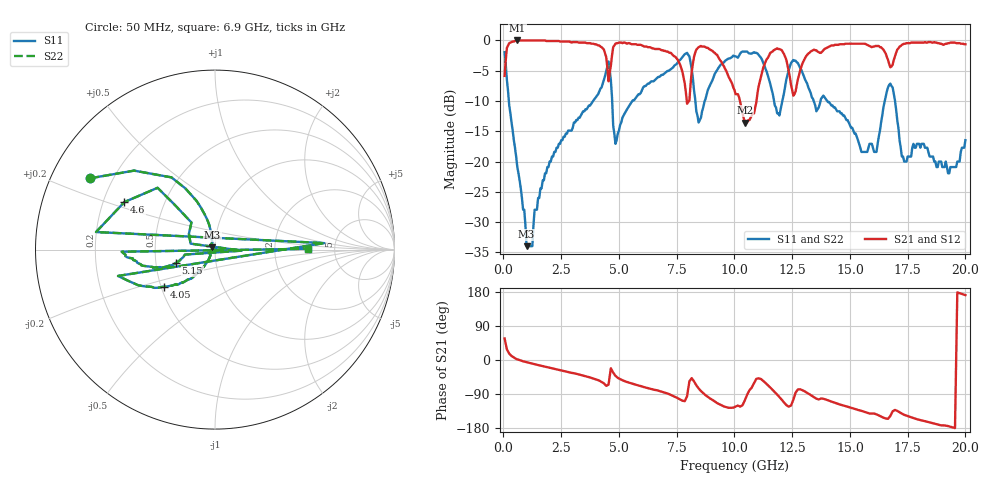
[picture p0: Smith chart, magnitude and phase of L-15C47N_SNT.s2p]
# MHZ S MA R 50
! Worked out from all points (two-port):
!   400 points, 50 MHz to 20 GHz, reference 50 ohm
!   highest |S21| = 0.00 dB at 600 MHz (marker M1); lowest = -13.6 dB at 10.45 GHz (marker M2)
!   |S21| within 3 dB of the highest: 105.5 MHz to 4.457 GHz (4.352 GHz wide, 191 % of centre); 13.05 GHz to 16.63 GHz (3.581 GHz wide, 24.1 % of centre)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
!   lowest |S11| = -34.0 dB at 1 GHz (marker M3), VSWR 1.04, Z = 48.5 + j1.27 ohm
!   |S11| at or under -10 dB: 234 MHz to 3.881 GHz (3.647 GHz wide, 177 % of centre); 14.02 GHz to 16.51 GHz (2.492 GHz wide, 16.3 % of centre); 16.95 GHz to end of sweep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
!   |S22| runs from -34.0 to -1.8 dB; largest |S21 - S12| = 0
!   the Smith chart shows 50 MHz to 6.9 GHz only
!   S11 on the Smith chart (normalised r, x): 50 MHz: 0.12, +0.26; 4.05 GHz: 0.52, -0.25; 4.6 GHz: 0.29, +0.23; 5.15 GHz: 0.64, -0.10; 6.9 GHz: 3.17, +0.04
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50  0.8 150.2  0.51 56.8  0.51 56.8  0.8 150.2
600  0.09 103.3  1 1.8  1 1.8  0.09 103.3
1000  0.02 139.3  1 -5.9  1 -5.9  0.02 139.3
3400  0.25 -133.8  0.96 -40.2  0.96 -40.2  0.25 -133.8
4050  0.35 -143.6  0.92 -52.0  0.92 -52.0  0.35 -143.6
4450  0.56 -164.8  0.73 -68.2  0.73 -68.2  0.56 -164.8
4500  0.61 3.4  0.59 -66.6  0.59 -66.6  0.61 3.4
4550  0.67 171.6  0.46 -65.0  0.46 -65.0  0.67 171.6
4600  0.57 152.3  0.54 -43.4  0.54 -43.4  0.57 152.3
5150  0.23 -161.2  0.95 -53.4  0.95 -53.4  0.23 -161.2
6700  0.5 -175.8  0.85 -80.8  0.85 -80.8  0.5 -175.8
6850  0.52 -178.7  0.83 -83.7  0.83 -83.7  0.52 -178.7
6900  0.52 0.5  0.83 -84.4  0.83 -84.4  0.52 0.5
6950  0.53 179.6  0.82 -85.2  0.82 -85.2  0.53 179.6
10050  0.74 117.2  0.36 -122.9  0.36 -122.9  0.74 117.2
10450  0.81 106.7  0.21 -106.5  0.21 -106.5  0.81 106.7
13350  0.34 21.9  0.82 -94.5  0.82 -94.5  0.34 21.9
16700  0.43 71.1  0.64 -151.5  0.64 -151.5  0.43 71.1
19550  0.09 -5.4  0.96 -179.7  0.96 -179.7  0.09 -5.4
19600  0.09 -6.6  0.95 -0.6  0.95 -0.6  0.09 -6.6
19650  0.1 -7.9  0.95 178.5  0.95 178.5  0.1 -7.9
20000  0.15 3.2  0.93 171.2  0.93 171.2  0.15 3.2
